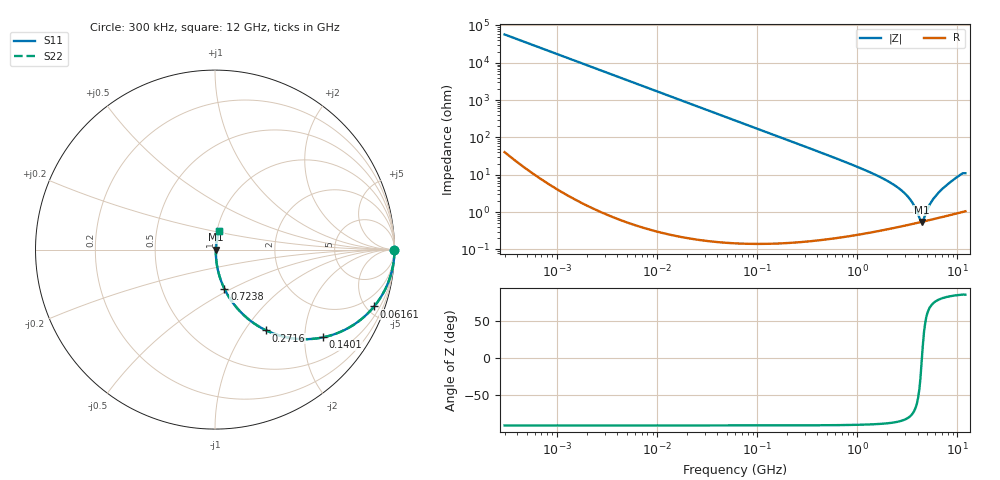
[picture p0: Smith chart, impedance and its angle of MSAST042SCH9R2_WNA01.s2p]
! MSAST042SCH9R2_WNA01  S-PARAMETER MODEL  ( General Type )
! Model Generated by TAIYO YUDEN Corporation (http://www.ty-top.com)
! Version 1.0
! TAIYO YUDEN Control No. 150820
! Copyright(c) 2015 TAIYO YUDEN CO.,LTD. All Rights Reserved.
! Product Description (link to TY-COMPAS)
! https://ds.yuden.co.jp/TYCOMPAS/or/detail?pn=MSAST042SCH9R2BWNA01&u=M
! Products Name : Multilayer Ceramic Capacitors
! Characteristics :
!  Capacitance : 9.2 pF , Rated Voltage : 25V , TCC : CH / C0H
!  Case Size : 0.4 x 0.2 / 0.016 x 0.008 [mm/inch] , Thickness : 0.2 / 0.008 [mm/inch]
!  (Conditions: Temperature = 25 degC , DC Bias Current/Voltage = 0A / 0V)
! External Node Assignments :
!  1  o---| |---o  2
! GND o---------o GND
! Frequency Range : 0.3MHz  -  12000MHz  [ 401 STEP ]
# MHz S RI R 50
! Freq[MHz].  S11 Real  S11 Imag  S21 Real  S21 Imag  S12 Real  S12 Imag  S22 Real  S22 Imag
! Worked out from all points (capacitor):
!   401 points, 300 kHz to 12 GHz, reference 50 ohm
!   read as one part in series: C = 9.24 pF near 316.3 kHz
!   lowest |Z| = 549 mohm at 4.385 GHz (marker M1)
!   series resonance near 4.411 GHz, so ESL is about 140 pH
!   S11 on the Smith chart (normalised r, x): 300 kHz: open; 61.61 MHz: 1.00, -5.59; 140.1 MHz: 1.00, -2.46; 271.6 MHz: 1.00, -1.26; 723.8 MHz: 1.00, -0.46; 12 GHz: 1.02, +0.22
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0.3  1 -0.00174  4.26e-06 0.00174  4.26e-06 0.00174  1 -0.00174
1.769972  0.9999 -0.0103  0.000107 0.0103  0.000107 0.0103  0.9999 -0.0103
10.44266  0.9963 -0.0604  0.00367 0.0604  0.00367 0.0604  0.9963 -0.0604
26.39317  0.977 -0.1497  0.023 0.1497  0.023 0.1497  0.977 -0.1497
60  0.8917 -0.3105  0.1083 0.3105  0.1083 0.3105  0.8917 -0.3105
61.61074  0.8864 -0.317  0.1136 0.317  0.1136 0.317  0.8864 -0.317
91.67136  0.779 -0.4145  0.221 0.4145  0.221 0.4145  0.779 -0.4145
140.0606  0.6015 -0.489  0.3985 0.489  0.3985 0.489  0.6015 -0.489
271.6094  0.2859 -0.4506  0.7141 0.4506  0.7141 0.4506  0.2859 -0.4506
353.9943  0.1904 -0.3909  0.8096 0.3909  0.8096 0.3909  0.1904 -0.3909
723.8279  0.0527 -0.219  0.9473 0.219  0.9473 0.219  0.0527 -0.219
2088.533  0.00759 -0.0634  0.9924 0.0634  0.9924 0.0634  0.00759 -0.0634
2650.866  0.00575 -0.0412  0.9942 0.0412  0.9942 0.0412  0.00575 -0.0412
3190.978  0.00516 -0.0256  0.9948 0.0256  0.9948 0.0256  0.00516 -0.0256
3547.679  0.00508 -0.0171  0.9949 0.0171  0.9949 0.0171  0.00508 -0.0171
4158.869  0.00529 -0.00472  0.9947 0.00472  0.9947 0.00472  0.00529 -0.00472
4385.161  0.00545 -0.000428  0.9946 0.000428  0.9946 0.000428  0.00545 -0.000428
4623.766  0.00564 0.00372  0.9944 -0.00372  0.9944 -0.00372  0.00564 0.00372
5565.855  0.00667 0.0187  0.9933 -0.0187  0.9933 -0.0187  0.00667 0.0187
6524.734  0.00808 0.0328  0.9919 -0.0328  0.9919 -0.0328  0.00808 0.0328
9454.42  0.015 0.0774  0.985 -0.0774  0.985 -0.0774  0.015 0.0774
12000  0.022 0.1062  0.978 -0.1062  0.978 -0.1062  0.022 0.1062
